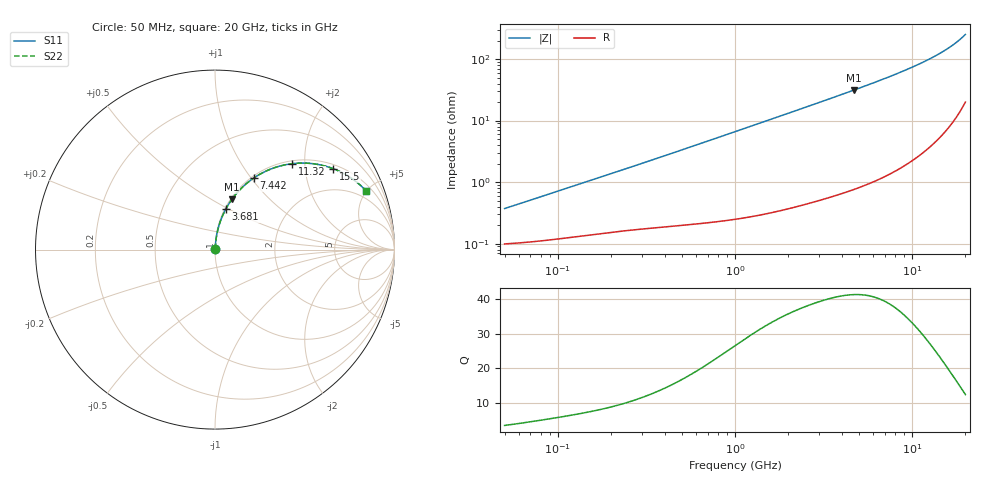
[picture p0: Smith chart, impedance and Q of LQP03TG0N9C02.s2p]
!Murata Part Number: LQP03TG0N9C02
!These Parameters are Measured in Series Mode Connection
!  o--[Z]--o
!Port1  Port2
!  o-------o
!Freq. Start=50[MHz] Stop=20[GHz], 401[Steps]
# Hz S RI R 50
!Freq.(Hz) S11(Real) S11(Imag) S21(Real) S21(Imag) S12(Real) S12(Imag) S22(Real) S22(Imag)
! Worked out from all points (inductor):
!   401 points, 50 MHz to 20 GHz, reference 50 ohm
!   read as one part in series: L = 1.13 nH near 51.52 MHz
!   highest Q = 41.2 at 4.678 GHz (marker M1), where L = 1.06 nH
!   S11 on the Smith chart (normalised r, x): 50 MHz: 1.00, +0.01; 3.681 GHz: 1.01, +0.49; 7.442 GHz: 1.03, +1.03; 11.32 GHz: 1.06, +1.73; 15.5 GHz: 1.14, +2.82; 20 GHz: 1.40, +5.00
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5e7  0.001 0.00358  0.999 -0.00358  0.999 -0.00358  0.001 0.00358
5.470171e7  0.00102 0.00391  0.999 -0.00391  0.999 -0.00391  0.00102 0.00391
1.364002e8  0.00142 0.00945  0.9986 -0.00945  0.9986 -0.00945  0.00142 0.00945
3.721004e8  0.00244 0.0248  0.9976 -0.0248  0.9976 -0.0248  0.00244 0.0248
6.380365e8  0.00388 0.042  0.9961 -0.042  0.9961 -0.042  0.00388 0.042
1e9  0.00677 0.0653  0.9932 -0.0653  0.9932 -0.0653  0.00677 0.0653
1.714689e9  0.0157 0.1105  0.9843 -0.1105  0.9843 -0.1105  0.0157 0.1105
2.728004e9  0.0354 0.1723  0.9646 -0.1723  0.9646 -0.1723  0.0354 0.1723
3.680849e9  0.0609 0.227  0.9391 -0.227  0.9391 -0.227  0.0609 0.227
4.677679e9  0.0941 0.2802  0.9059 -0.2802  0.9059 -0.2802  0.0941 0.2802
5.944466e9  0.1453 0.3403  0.8547 -0.3403  0.8547 -0.3403  0.1453 0.3403
7.442007e9  0.2163 0.399  0.7837 -0.399  0.7837 -0.399  0.2163 0.399
8.264682e9  0.2591 0.4248  0.7409 -0.4248  0.7409 -0.4248  0.2591 0.4248
9.178299e9  0.309 0.448  0.691 -0.448  0.691 -0.448  0.309 0.448
1.019291e10  0.3662 0.4667  0.6338 -0.4667  0.6338 -0.4667  0.3662 0.4667
1.131968e10  0.4308 0.4788  0.5692 -0.4788  0.5692 -0.4788  0.4308 0.4788
1.334722e10  0.5456 0.4786  0.4544 -0.4786  0.4544 -0.4786  0.5456 0.4786
1.438523e10  0.6018 0.4684  0.3982 -0.4684  0.3982 -0.4684  0.6018 0.4684
1.550395e10  0.6592 0.4506  0.3408 -0.4506  0.3408 -0.4506  0.6592 0.4506
1.747767e10  0.7502 0.4045  0.2498 -0.4045  0.2498 -0.4045  0.7502 0.4045
1.940974e10  0.8244 0.3453  0.1756 -0.3453  0.1756 -0.3453  0.8244 0.3453
2e10  0.8439 0.3252  0.1561 -0.3252  0.1561 -0.3252  0.8439 0.3252
